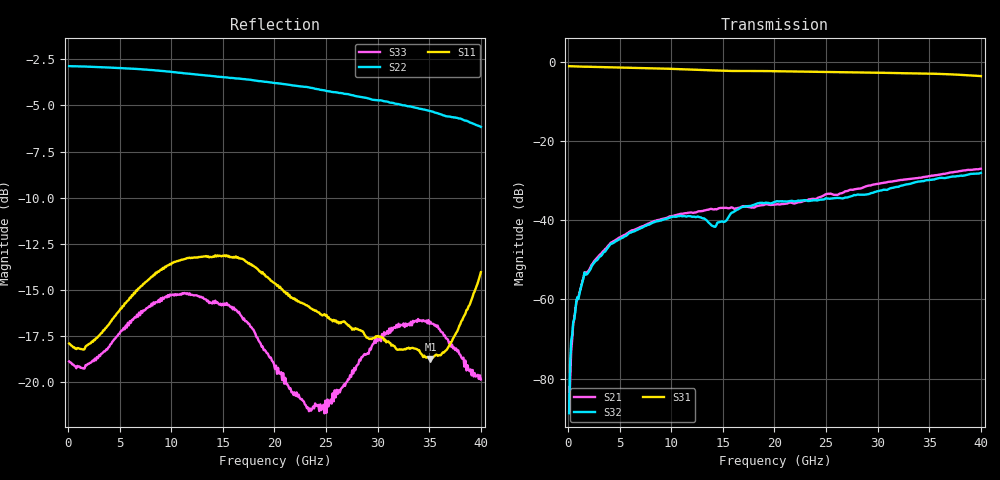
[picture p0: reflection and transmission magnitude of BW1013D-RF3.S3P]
!  3-Port S-parameters saved by WinCal
! VAR MeasName=S-Parameters (CALIBRATED_DATA) read from VNA (N5245A)
! VAR MeasDate=12/26/2016 18:42:19
! VAR NAME=158306_25-RF3
! VAR FILENAME=158306_25-RF3.S3P
! VAR DATE=12/26/2016 18:42:19
! VAR PHYS_PORTS=1,2,3
# Hz S RI R 50
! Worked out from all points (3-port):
!   401 points, 100 MHz to 40 GHz, reference 50 ohm
!   strongest paths, dB at 100 MHz, 10.07 GHz, 20.05 GHz, 30.02 GHz, 40 GHz:
!     S31: -1.1, -1.8, -2.4, -2.8, -3.6
!     S32: -88.8, -39.2, -35.4, -32.7, -28.1
!     S21: -88.2, -39.0, -36.1, -30.9, -27.0
!   lowest |S11| = -18.7 dB at 35.11 GHz (marker M1), VSWR 1.26, Z = 42.2 + j7.35 ohm
!   |S11| at or under -10 dB: start of sweep to end of sweep
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1e8  0.1273 -0.00567  -4.66e-05 7.14e-05  0.8758 -0.0121
     -3.14e-05 -2.28e-05  -0.7178 0.00286  5.25e-05 6.12e-05
     0.8763 -0.0119  -3.1e-05 1.9e-05  0.1138 -0.00494
6.985e8  0.1196 -0.0308  -0.000264 0.000637  0.8664 -0.0739
         -0.000246 0.00067  -0.7169 0.0175  -0.000195 0.000634
         0.8671 -0.074  -0.000167 0.00068  0.107 -0.0275
1.39675e9  0.1108 -0.0532  -0.000234 0.0017  0.8524 -0.1384
           -0.000189 0.00168  -0.7157 0.0341  -0.000108 0.00161
           0.8529 -0.1386  -7.27e-05 0.00166  0.0986 -0.047
4.18975e9  0.0677 -0.1301  0.00187 0.00489  0.7621 -0.3742
           0.0019 0.00488  -0.7044 0.0987  0.00227 0.00449
           0.7626 -0.3743  0.00226 0.00451  0.0586 -0.1129
1.157125e10  -0.1179 -0.1824  0.0113 0.00482  0.2717 -0.7495
             0.0114 0.00475  -0.6365 0.2543  0.0113 0.000498
             0.2718 -0.7498  0.0112 0.000476  -0.1038 -0.1401
1.416475e10  -0.1568 -0.1526  0.0138 0.00216  0.0698 -0.771
             0.0135 0.00197  -0.603 0.3019  0.00852 -0.00106
             0.0707 -0.7709  0.0082 -0.000877  -0.1239 -0.107
2.005e10  -0.1741 -0.0628  0.0147 -0.0048  -0.3483 -0.6721
          0.0149 -0.00474  -0.5074 0.3997  0.014 -0.00939
          -0.3481 -0.6734  0.0142 -0.00935  -0.1012 -0.0398
2.832925e10  -0.1375 -0.0164  0.015 -0.02  -0.7092 -0.1737
             0.0149 -0.0202  -0.322 0.4979  0.00385 -0.0204
             -0.7103 -0.1739  0.00398 -0.0205  -0.0555 -0.1003
3.511225e10  -0.0775 0.0859  -0.0076 -0.0354  -0.6148 0.3444
             -0.00779 -0.0351  -0.1354 0.5253  -0.0166 -0.0273
             -0.6158 0.3445  -0.0169 -0.0274  -0.0958 -0.1101
4e10  0.1367 0.1444  -0.0353 -0.0274  -0.2927 0.5867
      -0.0353 -0.0271  0.0116 0.4914  -0.0372 -0.0136
      -0.2938 0.5876  -0.0371 -0.0134  -0.0482 -0.0897
